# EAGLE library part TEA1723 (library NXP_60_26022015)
Switch mode power supply controller The TEA1723 is a small and low cost module Switched Mode Power Supply (SMPS) controller IC for power applications (up to 11 W) and operates directly from the rectified universal mains input. The device includes a high voltage power switch (700 V) and has been optimized for flyback converter topologies to provide high-efficiency over the entire load range with ultra-low power consumption in the no-load condition. It provides a circuit for start-up directly from the rectified mains voltage without any external bleeder circuits. The converter operates as a regulated voltage source from no-load up to the maximum output current and operates as current source that delivers the maximum current over a broad output voltage range. Using the TEA1723, a low power converter can be built at minimum cost and with the minimum number of external components. The controller regulates the output voltage with primary-side sensing which eliminates the need for an additional secondary feedback circuitry and simplifies the design. At higher power levels, a frequency and current control mode is used. It operates with burst mode control at low power levels and no-load condition. The burst mode minimizes audible noise and provides an energy saver state which reduces the power consumption in no-load condition. The Burst mode frequency of 1750 Hz enables no-load power consumption AAL Eindhoven MK
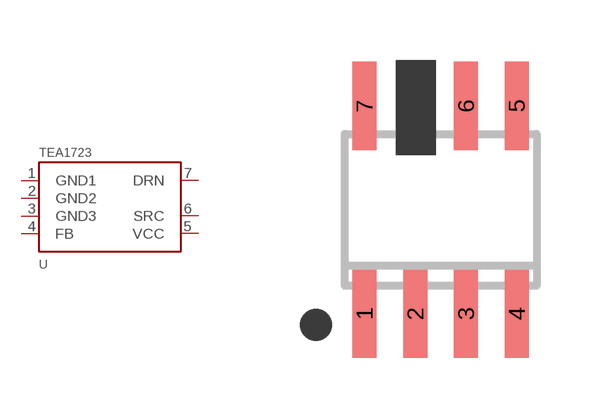
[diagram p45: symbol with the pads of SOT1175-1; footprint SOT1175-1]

Designator prefix U

## TEA1723 (12NC: 9352 968 88118)  [SOT1175-1]
1  GND1  pwr
2  GND2  pwr
3  GND3  pwr
4  FB
5  VCC  pwr
6  SRC  in
7  DRN  out

## Footprint SOT1175-1 (pad centres in mm)
SOT1175-1 SO7: plastic small outline package; 7 leads; body width 3.9 m JEDEC: --- IEC: ---
smd 0.6 x 2.2: 1 -1.905,-2.6; 2 -0.635,-2.6; 3 0.635,-2.6; 4 1.905,-2.6; 5 1.905,2.6; 6 0.635,2.6; 7 -1.905,2.6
